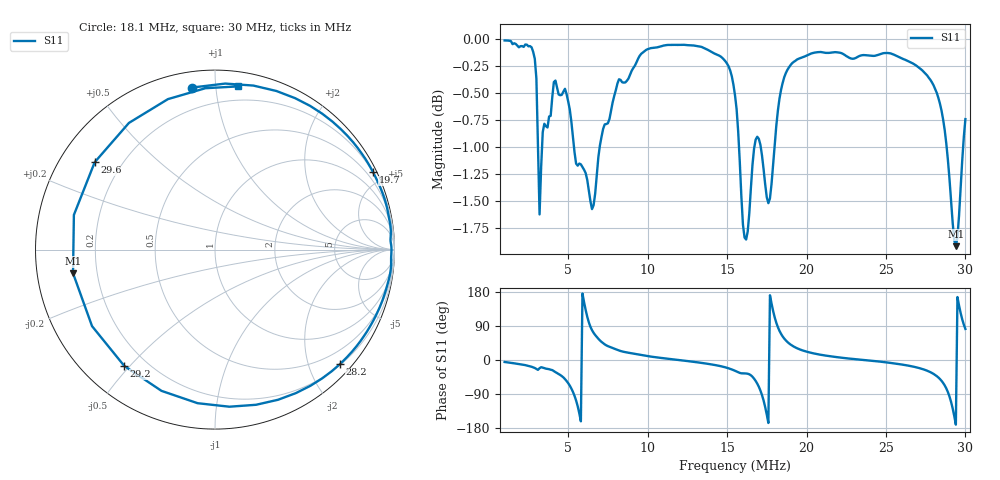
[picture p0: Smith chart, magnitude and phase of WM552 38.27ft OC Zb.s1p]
!Created via Zplots "Save as S1P" button
!Original data file:  $remote$.s1p
!Transmission line transform:  None
# MHZ S MA R 50
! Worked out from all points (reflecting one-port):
!   291 points, 1 MHz to 30 MHz, reference 50 ohm
!   lowest |S11| = -1.9 dB at 29.4 MHz (marker M1), VSWR 9.09, Z = 5.53 - j4.08 ohm
!   phase of S11 starts at -5 deg and turns -993 deg over the sweep
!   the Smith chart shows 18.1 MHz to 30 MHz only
!   S11 on the Smith chart (normalised r, x): 18.1 MHz: 0.08, +0.86; 19.7 MHz: 0.19, +4.32; 28.2 MHz: 0.22, -2.55; 29.2 MHz: 0.12, -0.48; 29.6 MHz: 0.10, +0.32; 30 MHz: 0.10, +1.15
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1  0.9986 -5.2
3.3  0.8726 -18.9
4.7  0.9456 -46.0
5.5  0.8756 -107.0
5.7  0.8757 -140.5
5.9  0.8725 175.4
6.1  0.8669 132.2
6.3  0.8513 99.5
7  0.8929 51.6
8.3  0.9574 23.7
11.9  0.9939 0.2
15.5  0.9419 -28.4
16.7  0.8897 -49.2
17.3  0.8704 -107.0
17.7  0.8438 170.9
17.9  0.8753 129.2
18.1  0.9119 98.2
18.6  0.9603 56.5
19.2  0.9761 35.4
19.7  0.9804 26.0
22.8  0.9796 3.3
26.4  0.9768 -14.8
28.2  0.9442 -42.6
28.7  0.9074 -67.2
29.2  0.8221 -127.9
29.4  0.8019 -170.5
29.6  0.8284 144.0
30  0.9183 82.0
